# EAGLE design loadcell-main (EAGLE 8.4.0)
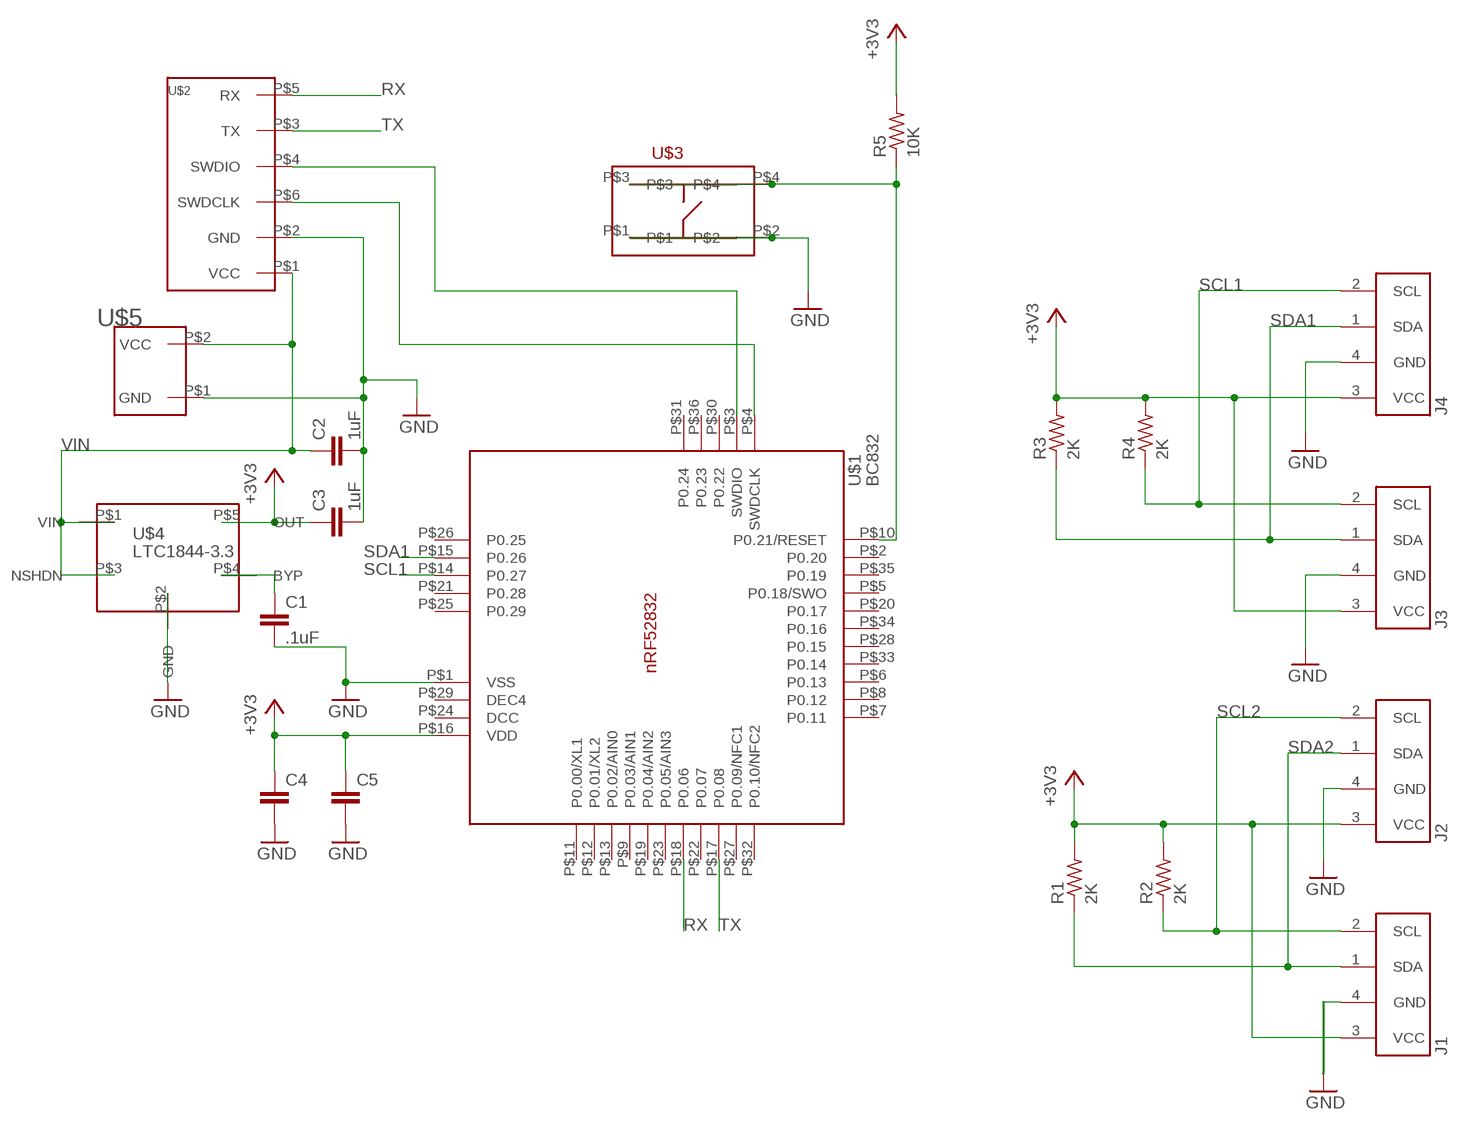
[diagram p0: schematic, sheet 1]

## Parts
C1  .1uF  CAPACITOR_0805_L  [RESC0805_L]
C2  1uF  CAPACITOR_0805_L  [RESC0805_L]
C3  1uF  CAPACITOR_0805_L  [RESC0805_L]
C4  CAPACITOR  [1206_MILL]
C5  CAPACITOR  [1206_MILL]
J1  TWI-MILLMAXRECV  [MILLMAX-22-004-40-001101_RECV]
J2  TWI-MILLMAXRECV  [MILLMAX-22-004-40-001101_RECV]
J3  TWI-MILLMAXRECV  [MILLMAX-22-004-40-001101_RECV]
J4  TWI-MILLMAXRECV  [MILLMAX-22-004-40-001101_RECV]
R1  2K  RESISTOR  [1206_MILL]
R2  2K  RESISTOR  [1206_MILL]
R3  2K  RESISTOR  [1206_MILL]
R4  2K  RESISTOR  [1206_MILL]
R5  10K  RESISTOR  [1206_MILL]
U$1  BC832  [FANSTEL_BC832]
U$2  TAGCONNECT_SWD_SERIAL  [TAG-CONNECT]
U$3  TACTILE_SWITCH_KMR7  [TACTILE_SWITCH_KMR7]
U$4  LTC1844-3.3  [TSOT-23-5]
U$5  JST-CONNECT-ACH-2  [JST-CONNECT-ACH-2]

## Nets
+3V3: C3.1 C4.1 C5.1 J1.3(VCC) J2.3(VCC) J3.3(VCC) J4.3(VCC) R1.2 R2.2 R3.2 R4.2 R5.2 U$1.P$16(VDD) U$4.P$5(OUT)
GND: C1.2 C2.2 C3.2 C4.2 C5.2 J1.4(GND) J2.4(GND) J3.4(GND) J4.4(GND) U$1.P$1(VSS) U$2.P$2(GND) U$3.P$1 U$3.P$2 U$4.P$2(GND) U$5.P$1(GND)
N$1: U$1.P$3(SWDIO) U$2.P$4(SWDIO)
N$2: U$1.P$4(SWDCLK) U$2.P$6(SWDCLK)
N$5: R5.1 U$1.P$10(P0.21/RESET) U$3.P$3 U$3.P$4
N$6: C1.1 U$4.P$4(BYP)
RX: U$1.P$18(P0.06) U$2.P$5(RX)
SCL1: J3.2(SCL) J4.2(SCL) R4.1 U$1.P$14(P0.27)
SCL2: J1.2(SCL) J2.2(SCL) R2.1
SDA1: J3.1(SDA) J4.1(SDA) R3.1 U$1.P$15(P0.26)
SDA2: J1.1(SDA) J2.1(SDA) R1.1
TX: U$1.P$17(P0.08) U$2.P$3(TX)
VIN: C2.1 U$2.P$1(VCC) U$4.P$1(VIN) U$4.P$3(NSHDN) U$5.P$2(VCC)
Unconnected: U$1.P$2(P0.20) U$1.P$5(P0.18/SWO) U$1.P$6(P0.13) U$1.P$7(P0.11) U$1.P$8(P0.12) U$1.P$9(P0.03/AIN1) U$1.P$11(P0.00/XL1) U$1.P$12(P0.01/XL2) U$1.P$13(P0.02/AIN0) U$1.P$19(P0.04/AIN2) U$1.P$20(P0.17) U$1.P$21(P0.28) U$1.P$22(P0.07) U$1.P$23(P0.05/AIN3) U$1.P$24(DCC) U$1.P$25(P0.29) U$1.P$26(P0.25) U$1.P$27(P0.09/NFC1) U$1.P$28(P0.15) U$1.P$30(P0.22) U$1.P$31(P0.24) U$1.P$32(P0.10/NFC2) U$1.P$33(P0.14) U$1.P$34(P0.16) U$1.P$35(P0.19) U$1.P$36(P0.23)

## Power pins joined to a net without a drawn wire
DEC4: U$1.P$29(DEC4)

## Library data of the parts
C1-C5 = sec:CAPACITOR: Generic chip capacitor
J1-J4 = sec:TWI-MILLMAX
R1-R5 = sec:RESISTOR
U$1 = sec:BC832
U$2 = sec:TAGCONNECT_SWD_SERIAL
U$3 = sec:TACTILE_SWITCH_KMR7
U$4 = sec:LTC1844-3.3
U$5 = sec:JST-CONNECT-ACH-2

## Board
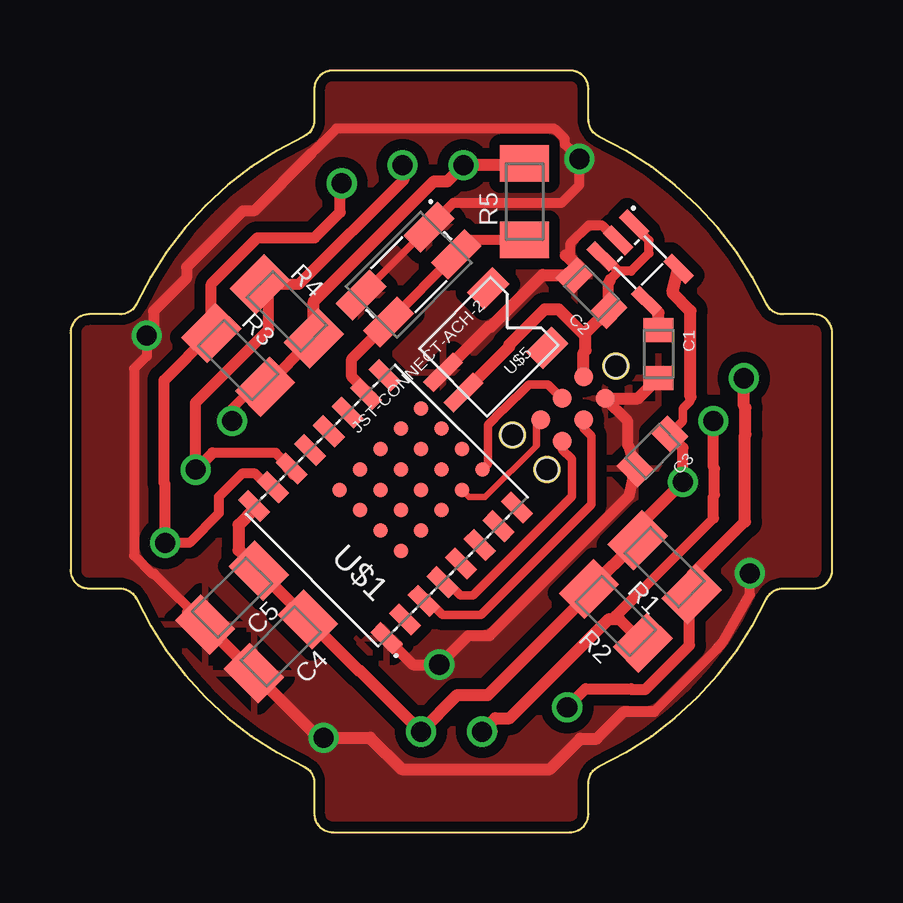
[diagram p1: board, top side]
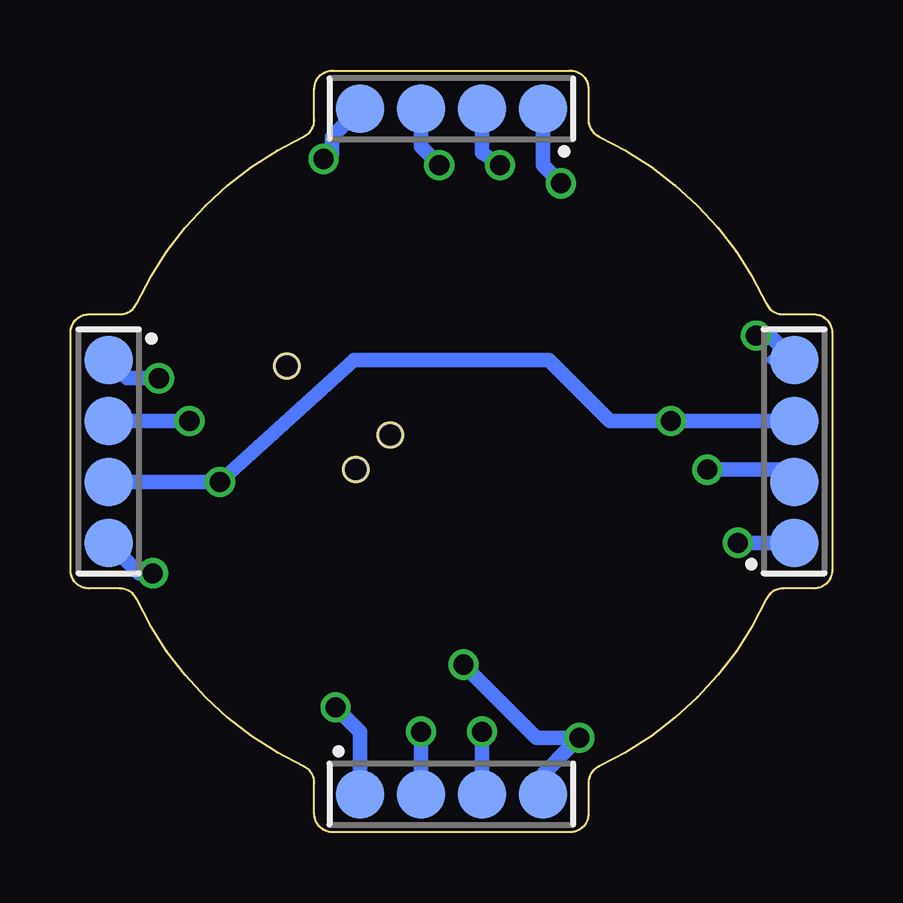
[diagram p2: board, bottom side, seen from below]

Size 31.75 x 31.75 mm. Coordinates in mm from the lower left corner, seen from the top.
Outline: 9.72,29 arc40 2.75,22.03 arc-65 2.06,21.59 0.76,21.59 arc90 0,20.83 0,10.92 arc90 0.76,10.16 2.06,10.16 arc-65 2.75,9.72 arc40 9.72,2.75 arc-65 10.16,2.06 10.16,0.76 arc90 10.92,0 20.83,0 arc90 21.59,0.76 21.59,2.06 arc-65 22.03,2.75 arc40 29,9.72 arc-65 29.69,10.16 30.99,10.16 arc90 31.75,10.92 31.75,20.83 arc90 30.99,21.59 29.69,21.59 arc-65 29,22.03 arc40 22.03,29 arc-65 21.59,29.69 21.59,30.99 arc90 20.83,31.75 10.92,31.75 arc90 10.16,30.99 10.16,29.69 arc-65 9.72,29
Copper layers (1*16): Top 0.035mm / dielectric 1.5mm / Bottom 0.035mm
Design rules "default *": minimum track width 6mil, minimum drill 0.35mm, track to track 18mil, track to pad 18mil, pad to pad 18mil, via to via 18mil, smd to smd 0mil, copper to edge 16mil, drill to drill 4mil, minimum pad ring 10mil, minimum via ring 8mil, stop-mask expansion 4mil, vias tented up to drill 0mil, thermal gap 18mil
bKeepout: area 20.9,5.4 to 26.4,10.8; area 5.4,5.4 to 10.8,10.8; area 5.4,20.9 to 10.8,26.4; area 20.9,20.9 to 26.4,26.4

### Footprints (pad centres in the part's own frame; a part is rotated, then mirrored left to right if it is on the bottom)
RESC0805_L = smd 1 x 1.25: 1 -1,0; 2 1,0
1206_MILL = smd 1.524 x 2.032: 1 -1.587,0; 2 1.587,0
MILLMAX-22-004-40-001101_RECV = smd 2.032 x 2.032: 1 -3.81,0; 2 -1.27,0; 3 1.27,0; 4 3.81,0
FANSTEL_BC832 = smd 1.3 x 0.6: P$1 0,-0.482; P$2 0,-1.582; P$3 0,-2.682; P$4 0,-3.782; P$5 0,-4.882; P$6 0,-5.982; P$7 0,-7.082; P$8 0,-8.182; P$9 7.8,-8.182; P$10 7.8,-7.082; P$11 7.8,-5.982; P$12 7.8,-4.882; P$13 7.8,-3.782; P$14 7.8,-2.682; P$15 7.8,-1.582; P$16 7.8,-0.482 | smd 0.6 x 0.6: P$17 2.15,-8.281; P$18 2.15,-7.081; P$19 2.15,-5.881; P$20 2.15,-4.681; P$21 2.15,-3.481; P$22 3.35,-8.281; P$23 3.35,-7.081; P$24 3.35,-5.881; P$25 3.35,-4.681; P$26 3.35,-3.481; P$27 4.55,-8.281; P$28 4.55,-7.081; P$29 4.55,-5.881; P$30 4.55,-4.681; P$31 4.55,-3.481; P$32 5.75,-8.281; P$33 5.75,-7.081; P$34 5.75,-5.881; P$35 5.75,-4.681; P$36 5.75,-3.481
TAG-CONNECT = smd 0.787 x 0.787: P$1 1.27,-0.635; P$2 1.27,0.635; P$3 2.54,-0.635; P$4 2.54,0.635; P$5 3.81,-0.635; P$6 3.81,0.635 | hole 0.998: 0,0; 5.08,1.016; 5.08,-1.016
TACTILE_SWITCH_KMR7 = smd 2 x 1: P$1 -2,-0.8; P$2 2,-0.8; P$3 -2,0.8; P$4 2,0.8
TSOT-23-5 = smd 1.3 x 0.5: P$1 -1.31,0.95; P$2 -1.31,0; P$3 -1.31,-0.95; P$4 1.31,-0.95; P$5 1.31,0.95
JST-CONNECT-ACH-2 = smd 1.75 x 0.6: P$1 4.2,-0.6; P$2 4.2,0.6 | smd 1.5 x 1: P$3 0.4,1.75; P$4 0.4,-1.75

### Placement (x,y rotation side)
C1  24.51,19.94 270 top
C2  21.72,22.48 135 top
C3  24.26,15.88 225 top
C4  8.76,7.75 225 top
C5  6.73,9.78 225 top
J1  15.88,1.59 0 bottom
J2  30.16,15.88 270 bottom
J3  15.88,30.16 180 bottom
J4  1.59,15.88 90 bottom
R1  24.77,11.05 135 top
R2  22.73,9.02 135 top
R3  6.98,19.68 315 top
R4  9.02,21.72 315 top
R5  18.92,26.29 90 top
U$1  12.83,7.75 135 top
U$2  22.73,19.43 225 top
U$3  14.1,23.24 225 top
U$4  23.75,23.75 315 top
U$5  18.92,21.72 225 top

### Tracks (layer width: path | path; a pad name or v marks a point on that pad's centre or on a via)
+3V3  (via drill 0.84)
  Top 0.305: 8.11,19.03 R3.2 | 25.58,14.66 v25.53,14.61
  Top 0.356: C3.1 25.53,17.15 25.53,17.67 25.85,17.98 25.85,18.14
  Top 0.406: v6.73,17.14 6.73,17.65 8.11,19.03
  Top 0.457: R3.2 R4.2 | v25.53,14.61 25.53,16.02 C3.1
  Top 0.508: 25.58,14.66 23.64,12.72 R1.2 R2.2 21.61,9.93 17.4,5.71 16.13,5.71 v14.61,4.19 12.06,6.73 12.02,6.73 C4.1 C5.1 7,11.76 7,12.81 7.65,13.47 U$1.P$16 | 25.85,18.14 25.85,21.73 25.09,22.49 U$4.P$5 | R4.2 10.14,22.13 15.15,27.14 15.71,27.14 v16.38,27.81 18.86,27.81 R5.2
  Bottom 0.61: J2.3 v25.53,14.61 19.94,19.68 11.81,19.68 9.27,17.14 v6.73,17.14 J4.3 | J1.3 v14.61,4.19 | J3.3 17.14,28.57 v16.38,27.81
GND  (via drill 0.84)
  Top 0.305: U$3.P$2 U$3.P$1 | 13.69,7.83 U$1.P$1
  Top 0.406: 15.35,25.73 U$3.P$1 15.95,26.23 20.46,26.23 21.21,26.98 v21.21,28.07 20.6,28.68 20.6,28.91 20.21,29.3 20.18,29.3 20.14,29.33 11.09,29.33 10.48,28.73 10.31,28.57 10.29,28.55 10.28,28.55 10.27,28.5 10.22,28.48 10.03,28.29 | U$1.P$1 13.34,7.75 | 4.85,9.16 C5.2 3.49,10.78 3.4,10.78 2.65,11.53 2.65,19.32 3.18,19.85 v3.18,20.7 | 24.33,5.04 26.92,7.63 27.18,7.94 28.32,9.91 v28.32,10.79 | C2.2 21.34,23.52 20.85,24.01 20.85,24.55 21.6,25.31 22.15,25.31 22.78,24.68 U$4.P$2
  Top 0.457: U$1.P$1 14.27,6.98 v15.37,6.98 16.58,8.2 17.47,8.2 23.3,14.03 C3.2 23.3,16.07 23.23,16.13 23.23,17.14 U$2.P$2 | 10.03,28.29 7.64,25.9 7.18,25.9 4.83,23.56 4.83,23.09 3.46,21.72 3.46,20.88 3.35,20.88 v3.18,20.7 | 21.93,3.89 23.07,5.04 24.33,5.04
  Top 0.508: C5.2 C4.2 10.33,3.94 v10.54,3.94 12.49,3.94 13.81,2.62 19.98,2.62 21.25,3.89 21.93,3.89 | U$2.P$2 23.66,18.08 C1.2 | U$5.P$1 17.43,21.08 17.52,21.08 19.67,23.23 20.97,23.23 C2.2 21.01,23.69 20.65,24.05 20.73,24.05
  Bottom 0.406: 2.52,19.68 J4.4
  Bottom 0.508: 12.06,2.41 J1.4 12.06,2.41 | 20.85,28.27 21.01,28.27 | 10.95,3.53 v10.54,3.94 | 12.06,2.41
  Bottom 0.61: v28.32,10.79 28.89,10.79 J2.4 | J3.4 20.85,28.99 20.85,28.27 | 21.01,28.27 v21.21,28.07 | J4.4 2.6,20.7 v3.18,20.7 | 12.06,2.41 10.95,3.53 | v10.54,3.94 12.32,3.94 v15.37,6.98
  pour Top: 8.51,-1.14 21.72,-1.14 32.89,10.03 32.89,21.21 21.72,32.39 10.03,32.39 -0.89,21.46 -0.89,8.25
N$1
  Top 0.305: 14.86,9.78 U$1.P$3
  Top 0.356: U$2.P$4 21.39,16.84 21.7,16.53 21.7,13.66 17.11,9.06 15.5,9.06 14.92,9.64 U$1.P$3
N$2
  Top 0.356: U$1.P$4 15.6,10.52 16.25,9.88 16.77,9.88 20.89,14 20.89,15.55 20.49,15.95 U$2.P$6
N$5
  Top 0.406: 12.57,18.18 U$1.P$10 | R5.1 16.69,24.7 U$3.P$3 U$3.P$4 12.57,20.59
  Top 0.457: U$1.P$10 12.32,18.4 11.72,18.99 11.72,19.73 12.57,20.59
N$6
  Top 0.508: C1.1 24.51,21.64 U$4.P$4
RX
  Top 0.279: 19.43,16.14 19.41,16.12 19.41,16.1 17.28,13.97 16.62,13.97 U$1.P$18
  Top 0.305: U$2.P$5 19.43,17.03 19.43,16.14
SCL1  (via drill 0.84)
  Top 0.406: 9.26,14.9 U$1.P$14 | U$1.P$14 9.05,15.16 | U$1.P$14 8.55,15.82 5.91,15.82
  Top 0.457: 9.08,15.16 U$1.P$14 | 5.91,15.82 v5.21,15.11 5.21,17.91 8.25,20.95 8.25,22.48 R4.1 9.52,22.84 13.91,27.23 13.91,27.74 v13.84,27.81
  Bottom 0.406: 1.84,14.86 J4.2
  Bottom 0.508: J4.2 2.1,15.11
  Bottom 0.61: J3.2 14.61,28.32 v13.84,27.81 | 2.1,15.11 v5.21,15.11
SCL2  (via drill 0.84)
  Top 0.305: 23.86,8.66 R2.1
  Top 0.406: 23.5,9.78 26.8,13.08
  Top 0.457: 26.8,13.08 26.8,14.02 26.84,14.06 26.84,15.15 26.8,15.19 v26.8,17.14 | 23.5,9.78 22.73,9.02 22.86,8.89 R2.1 | 17.57,4.19 v17.14,4.19
  Top 0.508: v17.14,4.19 17.7,4.75 18.3,4.75 22.44,8.89 22.86,8.89
  Bottom 0.61: J1.2 v17.14,4.19 | v26.8,17.14 J2.2
SDA1  (via drill 0.84)
  Top 0.406: v3.94,12.06 4.95,12.06 6.18,13.29 6.18,13.98 7.15,14.95 7.7,14.95 8.27,14.38 U$1.P$15
  Top 0.457: v3.94,12.06 3.94,14.52 3.89,14.57 3.89,18.84 R3.1 5.86,22.86 7.79,24.78 10.17,24.78 11.24,25.85 11.24,26.98 v11.3,27.05
  Bottom 0.61: J4.1 v3.94,12.06 | J3.1 12.06,27.81 v11.3,27.05
SDA2  (via drill 0.84)
  Top 0.305: 25.7,9.74 R1.1
  Top 0.457: v20.7,5.21 21.47,5.98 23.37,5.98 23.39,5.95 23.96,5.95 25.8,7.79 25.8,9.84 R1.1 25.89,10.73 28.11,12.95
  Top 0.508: v28.07,18.92 28.07,17.77 28.14,17.7 28.14,16.59 28.11,16.57 28.11,12.95
  Bottom 0.508: 29.66,19.18 J2.1
  Bottom 0.61: J1.1 19.68,4.19 v20.7,5.21 | J2.1 29.4,18.92 v28.07,18.92
TX
  Top 0.356: U$2.P$3 19.9,18.67 19.11,18.67 18.03,17.59 18,17.59 17.39,16.98 17.39,15.35 U$1.P$17
VIN
  Top 0.305: 16.47,18.32 U$5.P$2
  Top 0.381: U$4.P$1 23.21,25.57 23.63,25.15 | 23.63,25.15 23.86,24.92 | 21.93,24.29 21.92,24.28 U$4.P$3 22.21,24 | 22.83,23.38 23.37,23.38 24.11,24.13 24.11,24.67 23.63,25.15
  Top 0.406: 22.47,23.73 21.92,24.28 | U$4.P$3 22.21,24 22.83,23.38 22.49,23.05 22.49,22.99
  Top 0.457: C2.1 22.42,22.92 22.49,22.99 22.49,23.05
  Top 0.508: 21.46,19.06 U$2.P$1 21.39,19.99 21.47,20.08 21.47,20.82 | U$5.P$2 18.28,20.23 18.28,20.32 19.76,21.79 20.35,21.79 21.32,20.82 21.47,20.82 | 21.47,20.82 C2.1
